TYPE ST_CrossHmiData :
STRUCT
	bInCommissioning			: BOOL;		// command signal commissioning mode (on rising edge)
	bInAutomatic				: BOOL;		// command signal automatic mode (on rising edge)
	bInAutomaticActive			: BOOL;		// command signal automatic active mode (on rising edge) -> traffic lights H1/2 and V1/2 alternate 
	bInAutomaticStandBy			: BOOL;		// command signal automatic stand by mode (on rising edge) -> on all traffic lights the yellow light blinks
	bOutCommissioningMode		: BOOL;		// status signal commissioning mode active
	bOutAutomaticMode			: BOOL;		// status signal automatic mode active
	sOutName					: STRING;	// crossing name
END_STRUCT
END_TYPE
